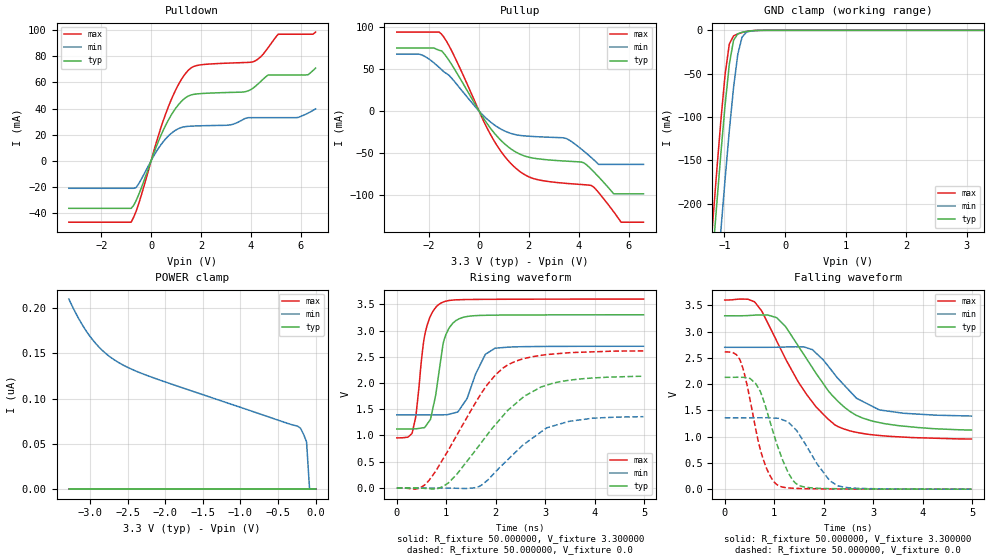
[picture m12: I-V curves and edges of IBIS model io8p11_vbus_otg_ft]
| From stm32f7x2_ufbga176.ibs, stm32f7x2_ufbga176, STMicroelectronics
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|   Model io8p11_vbus_otg_ft
[Model]  io8p11_vbus_otg_ft
Model_type I/O
Polarity   Non-Inverting
Enable   Active-Low
Vinl =   0.990000V
Vinh =   2.310000V
Vmeas =  1.650000V
Cref =   30.000000pF
Rref =   100.000000M
Vref =   0.0V
C_comp   3.304800pF   3.199300pF   3.429300pF
[Temperature Range]   25.000000   0.125000k   -40.000000
[Pullup Reference]   3.300000V   2.700000V   3.600000V
[Pulldown Reference]   0.0V   0.0V   0.0V
[POWER Clamp Reference]   3.300000V   2.700000V   3.600000V
[GND Clamp Reference]   0.0V   0.0V   0.0V
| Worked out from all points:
|   slope of the pulldown table from 0 to 0.495 V, typ, clamps not added: 20.9 ohm
|   slope of the pullup table from 0 to 0.495 V, typ, clamps not added: 22.6 ohm
|   GND clamp passes 1 mA (typ) near -0.61 V on its own axis
|   rising waveform, R_fixture 50.000000, V_fixture 3.300000: 20-80 % time 233ps typ, 350ps min, 206ps max; typ from 1.12 V to 3.3 V
|   rising waveform, R_fixture 50.000000, V_fixture 0.0: 20-80 % time 1.17ns typ, 982ps min, 1.02ns max; typ from 0 V to 2.13 V
|   falling waveform, R_fixture 50.000000, V_fixture 3.300000: 20-80 % time 1.03ns typ, 812ps min, 1.01ns max; typ from 3.3 V to 1.12 V
|   falling waveform, R_fixture 50.000000, V_fixture 0.0: 20-80 % time 451ps typ, 560ps min, 372ps max; typ from 2.13 V to 0 V
[Pulldown]
|Voltage   I(typ)   I(min)   I(max)
-3.3V     -36.41mA   -21.08mA   -47.04mA
-800mV    -36.41mA   -21.08mA   -47.04mA
-600mV    -30.48mA   -20.53mA   -38.65mA
700mV     31.4mA     19.11mA    41.71mA
1.2V      45.15mA    25.37mA    61.75mA
1.6V      50.35mA    26.5mA     71.06mA
3.1V      52.28mA    27.26mA    74.76mA
4.1V      55.7mA     33mA       75.81mA
4.7V      65.72mA    33mA       86.7mA
5.1V      65.72mA    33mA       96.91mA
6.3V      65.88mA    36.51mA    96.91mA
6.6V      70.94mA    39.72mA    98.51mA
[Pullup]
|Voltage   I(typ)   I(min)   I(max)
-3.3V     74.74mA    67.41mA    93.65mA
-2.3V     74.74mA    66.57mA    93.65mA
-1.5V     71.37mA    49mA       91.08mA
500mV     -22.07mA   -14mA      -30.03mA
1.6V      -50.64mA   -28.81mA   -70.96mA
3.5V      -59.53mA   -32.66mA   -85.92mA
4.2V      -61.44mA   -47.49mA   -87.46mA
4.5V      -69.06mA   -55.13mA   -88.4mA
4.8V      -78.22mA   -63.4mA    -96.84mA
5.4V      -98.3mA    -63.4mA    -119.6mA
5.7V      -98.3mA    -63.4mA    -132mA
6.6V      -98.3mA    -63.4mA    -132mA
[GND_clamp]
|Voltage   I(typ)   I(min)   I(max)
-3.3V     -2.319A    -2.398A    -2.292A
-1.2V     -265.6mA   -356.2mA   -227.3mA
-1.13V    -202.8mA   -293mA     -164.3mA
-1.06V    -142.3mA   -231.2mA   -104.3mA
-990mV    -86.15mA   -171.7mA   -51mA
-920mV    -39.05mA   -115.6mA   -15.71mA
-850mV    -11.4mA    -65.74mA   -6.366mA
-780mV    -4.046mA   -27.6mA    -4.153mA
-710mV    -2.285mA   -7.882mA   -2.591mA
-640mV    -1.291mA   -2.274mA   -1.367mA
-570mV    -618uA     -909.9uA   -567.3uA
3.28V     0A         0A         0A
[POWER_clamp]
|Voltage   I(typ)   I(min)   I(max)
-3.28V    0A         210.1nA    0A
-3.12V    0A         184.2nA    0A
-2.96V    0A         164.6nA    0A
-2.8V     0A         150.7nA    0A
-2.6V     0A         139nA      0A
-2.16V    0A         123.2nA    0A
-240mV    0A         69.7nA     0A
-200mV    0A         67.32nA    0A
-160mV    0A         60.72nA    0A
-120mV    0A         52.23nA    0A
-80mV     0A         0A         0A
0V        0A         0A         0A
[Ramp]
| variable   typ   min   max
dV/dt_r  1.25940/1.15705n   0.80064/0.97067n   1.56030/1.01780n
dV/dt_f  1.27500/1.00990n   0.76674/0.78518n   1.56937/1.00639n
R_load = 50.000000
[Rising Waveform]
R_fixture= 50.000000
V_fixture= 3.300000
V_fixture_min= 2.700000
V_fixture_max= 3.600000
|time   V(typ)   V(min)   V(max)
0s        1.124V     1.392V     954.4mV
310.3ps   1.126V     1.392V     1.044V
390.4ps   1.128V     1.392V     1.405V
570.6ps   1.161V     1.392V     2.938V
680.7ps   1.306V     1.392V     3.276V
880.9ps   2.394V     1.393V     3.516V
961ps     2.836V     1.395V     3.55V
1.131ns   3.138V     1.424V     3.58V
1.982ns   3.292V     2.661V     3.595V
4.985ns   3.3V       2.7V       3.599V
[Rising Waveform]
R_fixture= 50.000000
V_fixture= 0.0
V_fixture_min= 0.0
V_fixture_max= 0.0
|time   V(typ)   V(min)   V(max)
0s        345.2uV    194.4uV    641.6uV
560.6ps   -7.07mV    182.9uV    54.54mV
951ps     36.35mV    -1.04mV    577.8mV
1.662ns   807mV      26.94mV    1.736V
1.992ns   1.207V     303.6mV    2.152V
2.242ns   1.479V     539.1mV    2.344V
2.583ns   1.751V     841.6mV    2.468V
3.033ns   1.96V      1.148V     2.542V
3.964ns   2.096V     1.33V      2.594V
4.985ns   2.129V     1.359V     2.612V
[Falling Waveform]
R_fixture= 50.000000
V_fixture= 3.300000
V_fixture_min= 2.700000
V_fixture_max= 3.600000
|time   V(typ)   V(min)   V(max)
0s        3.3V       2.7V       3.599V
600.6ps   3.312V     2.7V       3.567V
750.8ps   3.315V     2.7V       3.386V
1.051ns   3.264V     2.701V     2.82V
1.491ns   2.717V     2.709V     2.033V
1.772ns   2.312V     2.655V     1.658V
2.232ns   1.726V     2.173V     1.221V
2.663ns   1.404V     1.73V      1.082V
3.123ns   1.267V     1.509V     1.022V
4.985ns   1.124V     1.392V     954.4mV
[Falling Waveform]
R_fixture= 50.000000
V_fixture= 0.0
V_fixture_min= 0.0
V_fixture_max= 0.0
|time   V(typ)   V(min)   V(max)
0s        2.129V     1.359V     2.612V
310.3ps   2.129V     1.359V     2.458V
460.5ps   2.117V     1.358V     1.948V
620.6ps   2.015V     1.358V     1.173V
840.8ps   1.523V     1.36V      407.4mV
1.081ns   786.8mV    1.349V     71.02mV
1.471ns   87.07mV    1.091V     14.42mV
1.872ns   17.89mV    473.4mV    7.003mV
2.292ns   8.087mV    61.52mV    4.071mV
4.985ns   345.2uV    194.4uV    641.6uV
